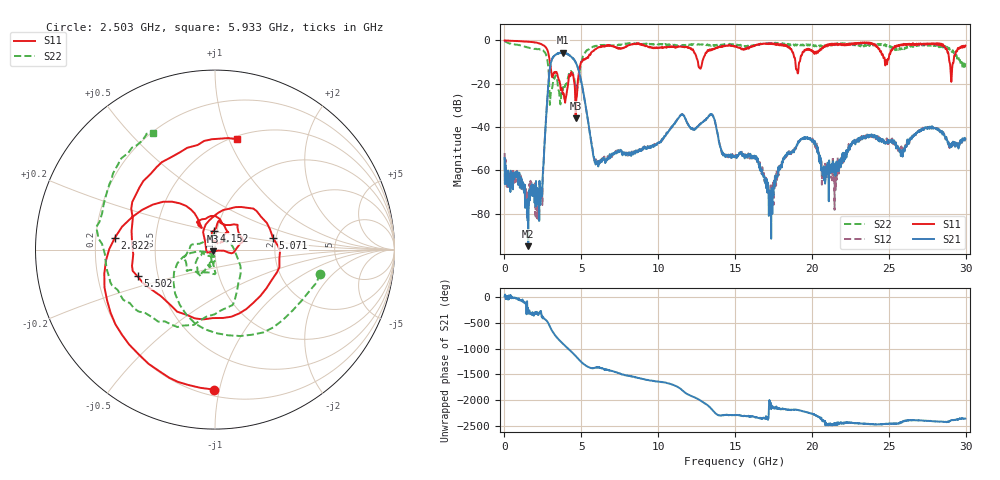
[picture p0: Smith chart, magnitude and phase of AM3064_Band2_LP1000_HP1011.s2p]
# Hz S DB R 50.0
!freq dBS11 angS11 dBS21 angS21 dBS12 angS12 dBS22 angS22
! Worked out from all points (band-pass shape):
!   1600 points, 10 MHz to 29.98 GHz, reference 50 ohm
!   highest |S21| = -5.63 dB at 3.777 GHz (marker M1); lowest = -94.9 dB at 1.547 GHz (marker M2)
!   |S21| within 3 dB of the highest: 3.094 GHz to 4.505 GHz (1.411 GHz wide, 37.1 % of centre)
!   lowest |S11| = -35.9 dB at 4.64 GHz (marker M3), VSWR 1.03, Z = 48.8 - j1.03 ohm
!   |S11| at or under -10 dB: 2.957 GHz to 5.017 GHz (2.06 GHz wide, 51.7 % of centre); 12.59 GHz to 12.87 GHz (280.8 MHz wide, 2.21 % of centre); 28.95 GHz to 29.21 GHz (255.6 MHz wide, 0.879 % of centre)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
!   |S22| runs from -29.7 to -0.3 dB; largest |S21 - S12| = 0.017
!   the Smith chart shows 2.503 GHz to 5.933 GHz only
!   S11 on the Smith chart (normalised r, x): 2.503 GHz: 0.24, -0.96; 2.822 GHz: 0.28, +0.05; 4.152 GHz: 0.96, +0.20; 5.071 GHz: 1.93, +0.27; 5.502 GHz: 0.38, -0.14; 5.933 GHz: 0.53, +1.07
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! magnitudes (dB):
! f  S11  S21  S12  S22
! 10 MHz  0.0  -54.3  -51.9  -0.3
! 1.547 GHz  -0.6  -94.9  -70.0  -3.3
! 2.278 GHz  -1.3  -64.8  -75.6  -4.0
! 2.503 GHz  -2.2  -61.0  -63.4  -4.4
! 2.822 GHz  -5.0  -23.5  -23.4  -10.6
! 3.777 GHz  -24.4  -5.6  -5.8  -23.1
! 4.152 GHz  -19.6  -6.6  -6.5  -16.6
! 4.64 GHz  -35.9  -10.4  -10.2  -21.8
! 5.015 GHz  -10.0  -19.7  -19.7  -9.7
! 5.071 GHz  -9.6  -21.8  -21.8  -8.5
! 5.502 GHz  -6.8  -40.3  -40.5  -4.0
! 5.933 GHz  -4.1  -57.3  -57.0  -2.7
! 10 GHz  -3.4  -47.1  -47.4  -1.8
! 13.43 GHz  -4.5  -34.1  -34.0  -2.5
! 15 GHz  -2.6  -53.7  -53.9  -1.8
! 16.34 GHz  -2.3  -54.7  -53.4  -2.4
! 17.35 GHz  -1.3  -91.5  -70.8  -1.3
! 18.27 GHz  -2.6  -53.4  -53.1  -1.8
! 19.99 GHz  -4.5  -46.6  -46.0  -1.9
! 20.95 GHz  -2.5  -61.7  -59.7  -2.1
! 25 GHz  -8.4  -47.4  -47.2  -2.3
! 29.98 GHz  -2.4  -45.5  -46.1  -10.5
